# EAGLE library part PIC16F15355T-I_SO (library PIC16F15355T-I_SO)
MCU 8-bit PIC RISC 14KB Flash 3.3V/5V 28-Pin SOIC W T/R Source: Datasheet
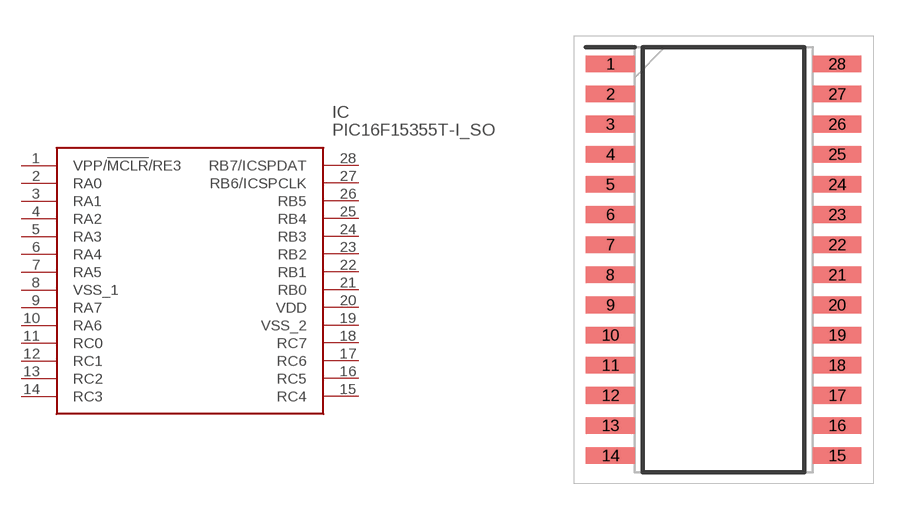
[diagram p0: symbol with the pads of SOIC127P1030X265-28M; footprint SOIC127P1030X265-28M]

Designator prefix IC

## PIC16F15355T-I_SO (Description: MCU 8-bit PIC RISC 14KB Flash 3.3V/5V 28-Pin SOIC W T/R; Height: 2.65mm; Manufacturer_Name: Microchip; Manufacturer_Part_Number: PIC16F15355T-I/SO; Mouser_Part_Number: 579-PIC16F15355TI/SO; Mouser_Price-Stock: https://www.mouser.co.uk/ProductDetail/Microchip-Technology/PIC16F15355T-I-SO?qs=8cKuZ6Ok2lZJ%2F9aGIYkbmQ%3D%3D)  [SOIC127P1030X265-28M]
1  VPP/!MCLR!/RE3
2  RA0
3  RA1
4  RA2
5  RA3
6  RA4
7  RA5
8  VSS_1
9  RA7
10  RA6
11  RC0
12  RC1
13  RC2
14  RC3
15  RC4
16  RC5
17  RC6
18  RC7
19  VSS_2
20  VDD
21  RB0
22  RB1
23  RB2
24  RB3
25  RB4
26  RB5
27  RB6/ICSPCLK
28  RB7/ICSPDAT

## Footprint SOIC127P1030X265-28M (pad centres in mm)
soic-28
smd 2.05 x 0.7: 1 -4.775,8.255; 2 -4.775,6.985; 3 -4.775,5.715; 4 -4.775,4.445; 5 -4.775,3.175; 6 -4.775,1.905; 7 -4.775,0.635; 8 -4.775,-0.635; 9 -4.775,-1.905; 10 -4.775,-3.175; 11 -4.775,-4.445; 12 -4.775,-5.715; 13 -4.775,-6.985; 14 -4.775,-8.255; 15 4.775,-8.255; 16 4.775,-6.985; 17 4.775,-5.715; 18 4.775,-4.445; 19 4.775,-3.175; 20 4.775,-1.905; 21 4.775,-0.635; 22 4.775,0.635; 23 4.775,1.905; 24 4.775,3.175; 25 4.775,4.445; 26 4.775,5.715; 27 4.775,6.985; 28 4.775,8.255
